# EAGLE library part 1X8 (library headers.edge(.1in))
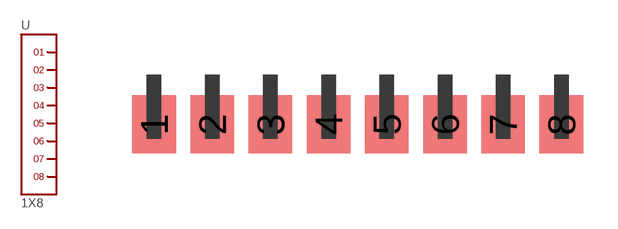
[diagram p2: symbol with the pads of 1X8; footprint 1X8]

Designator prefix -

## 1X8  [1X8]
1  1
2  2
3  3
4  4
5  5
6  6
7  7
8  8

## Footprint 1X8 (pad centres in mm)
smd 1.905 x 2.54: 1 0,-2.159; 2 2.54,-2.159; 3 5.08,-2.159; 4 7.62,-2.159; 5 10.16,-2.159; 6 12.7,-2.159; 7 15.24,-2.159; 8 17.78,-2.159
